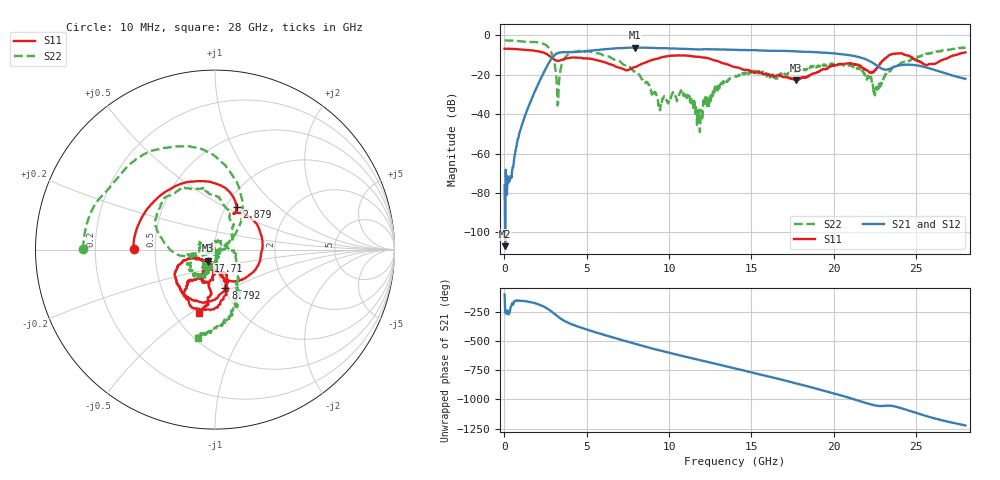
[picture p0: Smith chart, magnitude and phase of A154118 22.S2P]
!  2-Port S-parameters saved by WinCal
! VAR MeasName=S-Parameters (CALIBRATED_DATA) read from VNA (N5230A)
! VAR MeasDate=2015-9-10 14:36:03
! VAR NAME=A154118 22
! VAR FILENAME=A154118 22.S2P
! VAR DATE=2015-9-10 14:36:03
! VAR PHYS_PORTS=1,2
# Hz S DB R 50
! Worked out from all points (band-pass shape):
!   801 points, 10 MHz to 28 GHz, reference 50 ohm
!   highest |S21| = -6.24 dB at 7.952 GHz (marker M1); lowest = -106.9 dB at 44.99 MHz (marker M2)
!   |S21| within 3 dB of the highest: 3.193 GHz to 20.02 GHz (16.83 GHz wide, 145 % of centre); 20.03691 GHz to 20.06138 GHz (24.46 MHz wide, 0.122 % of centre)
!   lowest |S11| = -22.9 dB at 17.71 GHz (marker M3), VSWR 1.16, Z = 46 - j5.66 ohm
!   |S11| at or under -10 dB: 2.648 GHz to 23.4 GHz (20.75 GHz wide, 159 % of centre); 24.37 GHz to 27.4 GHz (3.037 GHz wide, 11.7 % of centre); 27.41069 GHz to 27.44782 GHz (37.13 MHz wide, 0.135 % of centre)
!   |S22| runs from -49.1 to -2.7 dB; largest |S21 - S12| = 0.008
!   S11 on the Smith chart (normalised r, x): 10 MHz: 0.38, +0.00; 2.879 GHz: 1.12, +0.57; 8.792 GHz: 1.02, -0.46; 17.71 GHz: 0.92, -0.11; 28 GHz: 0.66, -0.54
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1e7  -6.89 179.6  -76.15 -103.2  -76.19 143.0  -2.67 179.8
4.49875e7  -6.86 178.4  -106.93 104.7  -86.39 147.6  -2.68 178.9
1.304538e9  -7.42 132.7  -39.59 -160.4  -39.59 -160.3  -3.36 148.4
2.878975e9  -11.50 63.3  -11.70 109.4  -11.68 109.5  -9.42 64.8
3.263838e9  -13.00 62.8  -9.00 65.8  -8.98 65.9  -34.42 -135.4
3.683688e9  -11.89 53.0  -8.59 28.2  -8.57 28.5  -11.42 175.3
4.698325e9  -11.56 1.2  -8.29 -28.2  -8.25 -28.1  -7.97 131.6
6.30775e9  -14.46 -66.1  -6.95 -98.4  -6.88 -98.6  -10.76 84.9
7.952162e9  -16.13 -65.6  -6.24 -165.5  -6.22 -165.8  -18.84 34.3
8.791862e9  -13.03 -75.1  -6.39 162.2  -6.34 161.8  -25.19 1.7
9.351662e9  -11.83 -85.5  -6.61 142.2  -6.54 141.9  -35.77 -46.9
1.078615e10  -10.30 -118.7  -6.92 92.4  -6.82 91.7  -29.21 -167.6
1.190575e10  -11.09 -140.4  -7.22 56.0  -7.13 55.4  -43.48 95.0
1.274545e10  -12.72 -155.3  -7.15 27.4  -7.10 26.7  -29.17 -76.0
1.4005e10  -16.20 -162.0  -7.43 -15.1  -7.41 -15.7  -20.99 -98.0
1.771368e10  -22.85 -121.8  -8.16 -143.1  -8.17 -143.4  -18.59 -109.5
1.869332e10  -19.47 -95.8  -8.52 -178.2  -8.53 -178.6  -15.53 -109.6
2.15623e10  -15.18 -118.3  -11.20 67.1  -11.10 66.1  -16.16 -170.0
2.254195e10  -17.66 -77.8  -14.87 27.9  -14.84 27.3  -27.15 81.2
2.334666e10  -10.29 -84.4  -17.19 27.0  -17.09 25.8  -18.00 -11.7
2.565584e10  -15.10 -118.1  -16.43 -63.4  -16.44 -64.4  -9.54 -67.9
2.8e10  -8.72 -104.1  -22.13 -142.4  -22.18 -143.4  -6.03 -101.2
